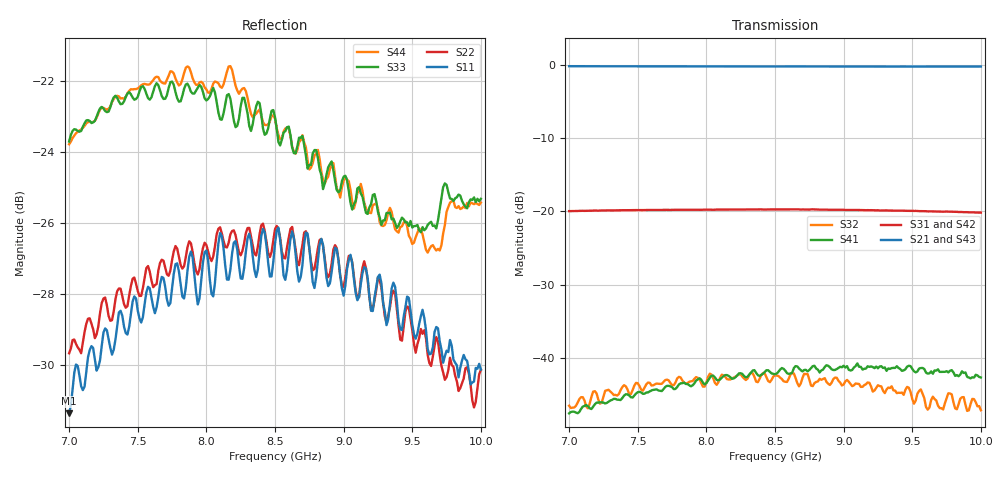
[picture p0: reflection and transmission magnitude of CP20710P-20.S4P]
! Amtery
! Email: info@amtery.com
! Phone: 886-2-2883-7839
! Model Number: CP20710P-20
! 4-port S-parameter measurement data for High Power Bi-Directional Coupler
! Frequency Range: 7 GHz to 10 GHz
! Port 1: Input
! Port 2: Output
! Port 3: Coupled Forward
! Port 4: Coupled Reverse
# Hz S dB R 50
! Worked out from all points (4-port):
!   241 points, 7 GHz to 10 GHz, reference 50 ohm
!   strongest paths, dB at 7 GHz, 7.75 GHz, 8.5 GHz, 9.25 GHz, 10 GHz:
!     S21: -0.2, -0.3, -0.3, -0.3, -0.3
!     S43: -0.3, -0.3, -0.3, -0.3, -0.3
!     S31: -20.0, -19.8, -19.8, -19.9, -20.2
!     S42: -20.0, -19.8, -19.8, -19.9, -20.2
!     S41: -47.5, -44.0, -42.2, -41.4, -42.7
!     S32: -46.5, -43.7, -42.3, -43.7, -47.1
!   lowest |S11| = -31.4 dB at 7 GHz (marker M1), VSWR 1.06, Z = 51.1 - j2.51 ohm
!   |S11| at or under -10 dB: start of sweep to end of sweep
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7e9  -31.36 -65.2  -0.23 -164.2  -19.99 -107.1  -48.29 -19.0
     -0.23 -164.4  -29.66 -101.2  -46.98 -44.0  -20.00 -112.4
     -19.99 -107.6  -46.52 -46.5  -23.71 -152.9  -0.25 123.1
     -47.55 -21.5  -19.99 -112.5  -0.25 123.1  -23.79 -142.2
7.65e9  -28.08 -117.2  -0.24 147.1  -19.82 -159.3  -44.59 -90.5
        -0.25 146.9  -27.34 -142.4  -43.87 -111.1  -19.84 -164.7
        -19.83 -159.7  -43.52 -110.9  -22.13 153.7  -0.29 67.2
        -44.42 -93.7  -19.84 -164.9  -0.29 67.2  -21.90 167.1
8.0625e9  -27.68 -153.1  -0.27 116.2  -19.79 167.8  -42.89 -131.1
          -0.27 116.0  -26.66 -168.3  -43.38 -148.5  -19.78 162.1
          -19.79 167.4  -43.40 -157.0  -22.33 120.5  -0.29 31.7
          -42.65 -134.5  -19.79 161.7  -0.30 31.7  -22.02 132.8
8.4375e9  -26.63 -176.0  -0.27 88.1  -19.74 137.9  -42.23 -168.0
          -0.27 88.0  -26.52 173.4  -43.23 170.8  -19.74 131.9
          -19.76 137.6  -42.63 162.7  -23.48 89.1  -0.28 -0.6
          -41.67 -171.9  -19.75 131.5  -0.27 -0.5  -23.25 100.3
8.8625e9  -27.06 148.3  -0.29 56.3  -19.78 103.6  -41.59 148.6
          -0.27 56.2  -26.99 146.4  -43.50 129.0  -19.78 97.5
          -19.79 103.3  -42.76 126.0  -24.88 57.2  -0.28 -37.2
          -41.22 148.0  -19.78 97.1  -0.27 -37.3  -24.89 59.1
9.275e9  -27.69 108.6  -0.30 25.4  -19.89 70.3  -41.31 109.7
         -0.27 25.2  -27.81 121.0  -44.15 95.6  -19.87 63.8
         -19.90 70.2  -43.88 89.8  -26.06 30.2  -0.27 -73.3
         -41.13 108.2  -19.89 63.7  -0.26 -73.3  -26.07 18.5
1e10  -30.13 31.6  -0.28 -29.0  -20.21 12.0  -42.50 43.8
      -0.27 -29.2  -30.13 84.0  -46.54 53.1  -20.18 5.0
      -20.19 11.5  -47.13 51.1  -25.32 -26.8  -0.30 -136.4
      -42.66 42.0  -20.19 4.8  -0.29 -136.4  -25.43 -54.7
